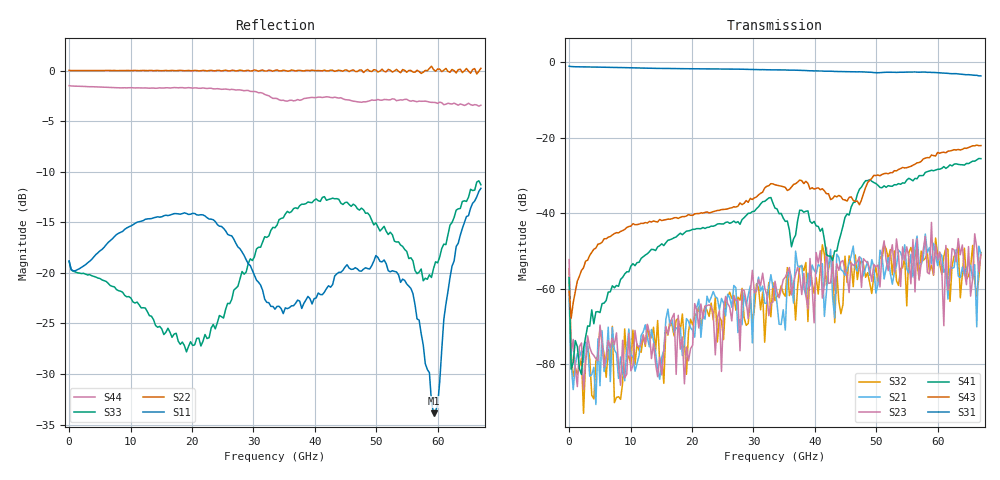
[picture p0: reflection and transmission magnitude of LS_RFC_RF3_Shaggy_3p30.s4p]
!Keysight Technologies,N5227A,US51270237,A.10.65.04
!Date: Tuesday, April 26, 2022 16:19:56
!Correction: S11(Full 4 Port(1,2,3,4))
!S12(Full 4 Port(1,2,3,4))
!S13(Full 4 Port(1,2,3,4))
!S14(Full 4 Port(1,2,3,4))
!S21(Full 4 Port(1,2,3,4))
!S22(Full 4 Port(1,2,3,4))
!S23(Full 4 Port(1,2,3,4))
!S24(Full 4 Port(1,2,3,4))
!S31(Full 4 Port(1,2,3,4))
!S32(Full 4 Port(1,2,3,4))
!S33(Full 4 Port(1,2,3,4))
!S34(Full 4 Port(1,2,3,4))
!S41(Full 4 Port(1,2,3,4))
!S42(Full 4 Port(1,2,3,4))
!S43(Full 4 Port(1,2,3,4))
!S44(Full 4 Port(1,2,3,4))
!S4P File: Measurements: <S11,S12,S13,S14>,
!<S21,S22,S23,S24>,
!<S31,S32,S33,S34>,
!<S41,S42,S43,S44>:
# Hz S  dB  R 50
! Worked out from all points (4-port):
!   201 points, 10 MHz to 67 GHz, reference 50 ohm
!   strongest paths, dB at 10 MHz, 16.76 GHz, 33.51 GHz, 50.25 GHz, 67 GHz:
!     S31: -1.1, -1.7, -2.1, -2.9, -3.7
!     S43: -60.6, -41.5, -32.5, -29.9, -22.1
!     S41: -57.1, -46.8, -38.7, -32.6, -25.6
!     S23: -52.3, -67.7, -58.0, -53.8, -51.0
!     S21: -62.7, -68.2, -59.8, -58.9, -50.7
!     S32: -54.7, -69.7, -63.2, -58.1, -50.4
!   lowest |S11| = -33.9 dB at 59.3 GHz (marker M1), VSWR 1.04, Z = 52.1 - j0.0624 ohm
!   |S11| at or under -10 dB: start of sweep to end of sweep
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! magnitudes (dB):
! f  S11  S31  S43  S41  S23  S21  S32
! 10 MHz  -18.8  -1.1  -60.6  -57.1  -52.3  -62.7  -54.7
! 1.015 GHz  -19.8  -1.3  -60.8  -73.7  -81.0  -80.2  -80.9
! 59.3 GHz  -33.9  -2.8  -24.8  -28.8  -56.3  -48.0  -56.4
! 64.32 GHz  -15.0  -3.3  -22.8  -27.3  -55.5  -56.5  -49.3
! 64.66 GHz  -14.4  -3.4  -22.9  -26.8  -58.9  -54.6  -57.5
! 66.33 GHz  -12.5  -3.5  -22.0  -25.9  -49.2  -70.1  -62.2
! 67 GHz  -11.6  -3.7  -22.1  -25.6  -51.0  -50.7  -50.4
